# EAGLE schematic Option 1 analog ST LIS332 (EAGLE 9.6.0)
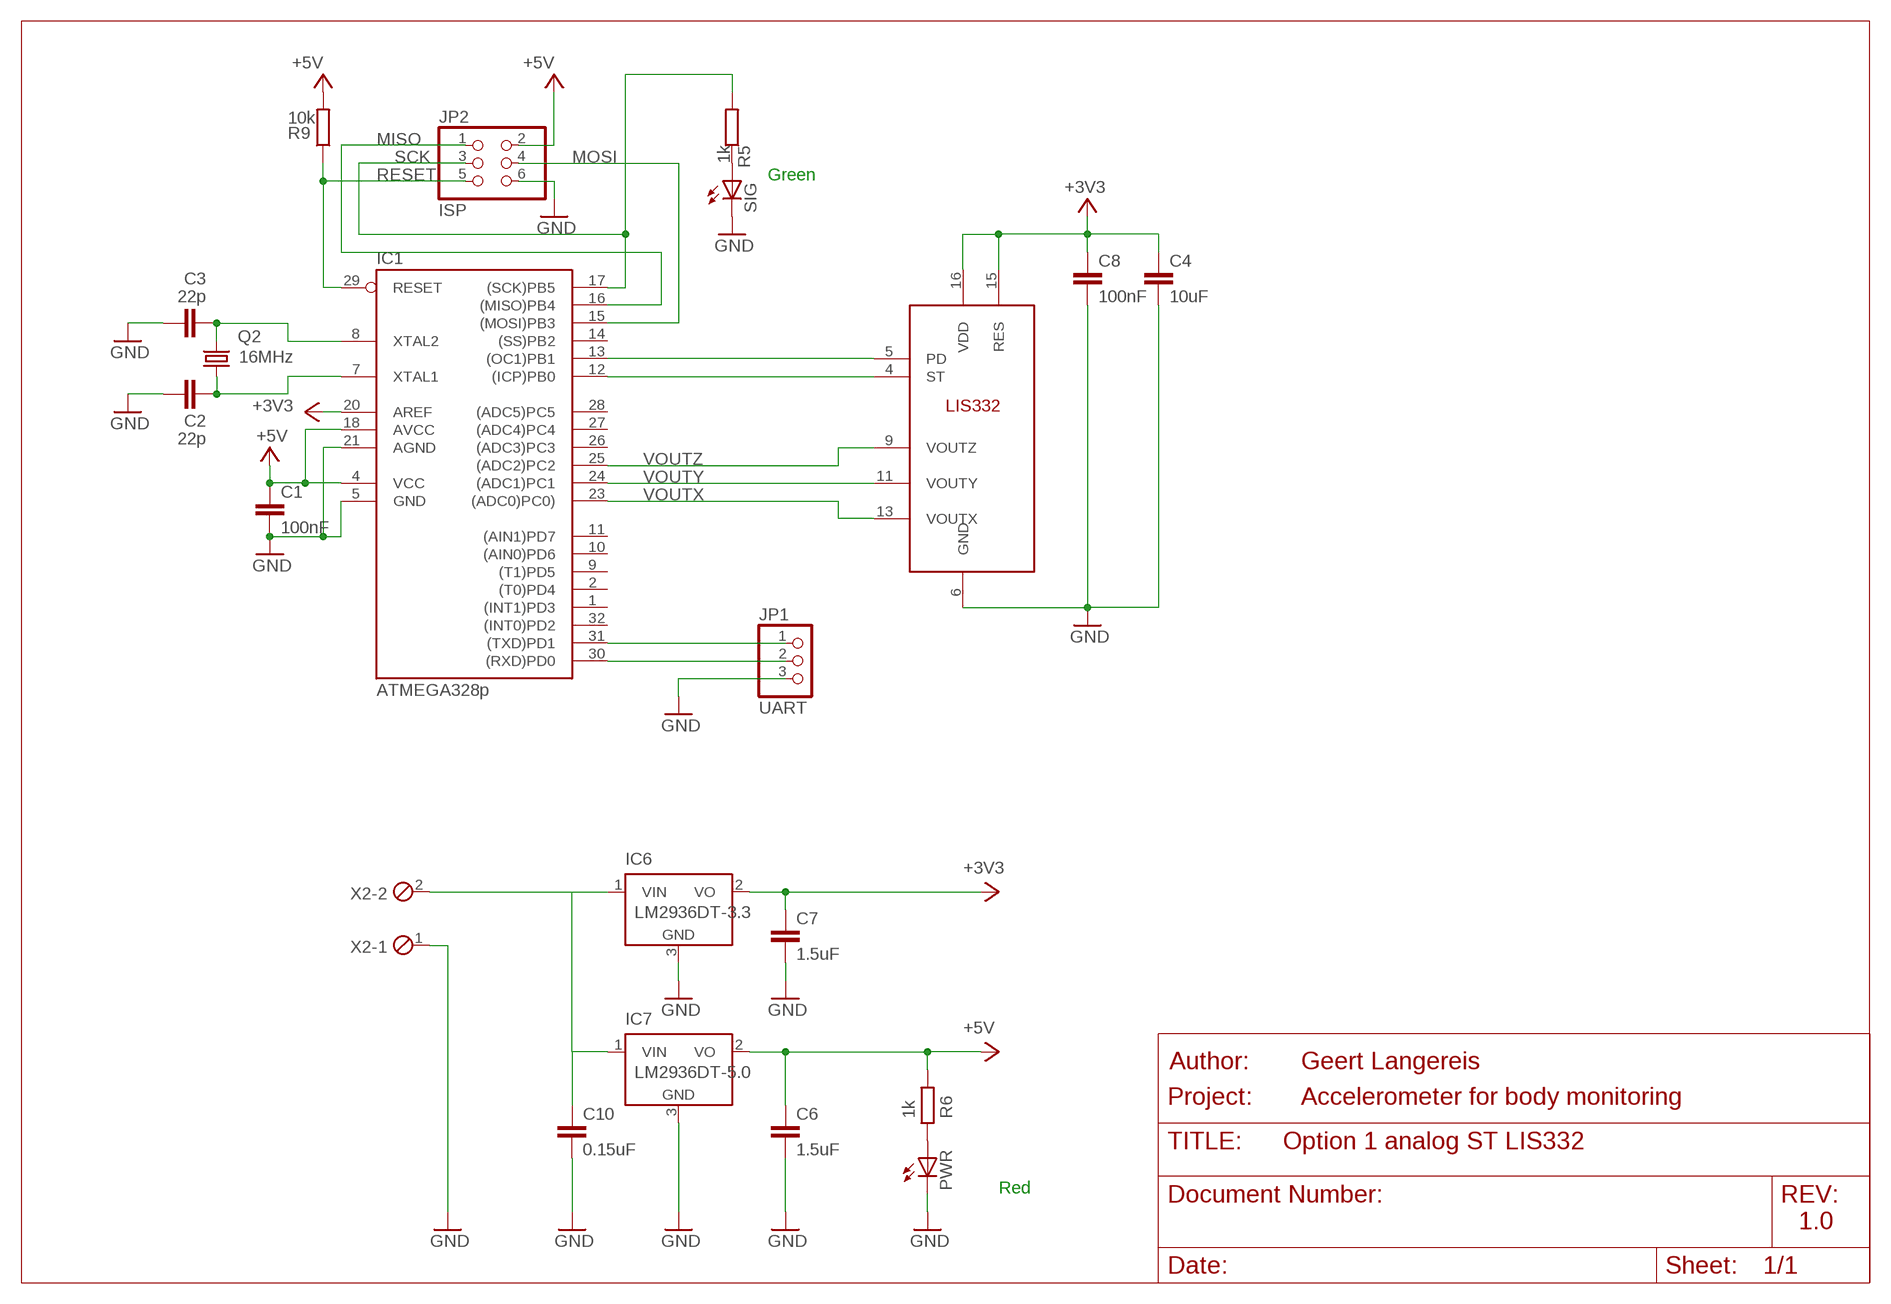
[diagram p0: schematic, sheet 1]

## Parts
C1  100nF  C5/3.5  [C5B3.5]
C2  22p  C2.5/2  [C2.5-2]
C3  22p  C2.5/2  [C2.5-2]
C4  10uF  C-EU050-030X075  [C050-030X075]
C6  1.5uF  C5/3.5  [C5B3.5]
C7  1.5uF  C5/3.5  [C5B3.5]
C8  100nF  C-EU050-030X075  [C050-030X075]
C10  0.15uF  C5/3.5  [C5B3.5]
IC1  ATMEGA328p  AT90S4433A  [TQFP32-08]
IC3  LIS332AR  [QFN-16]
IC6  LM2936DT-3.3  [TO252]
IC7  LM2936DT-5.0  [TO252]
JP1  UART  PINHD-1X3  [1X03]
JP2  ISP  PINHD-2X3  [2X03]
PWR  LED3MM  [LED3MM]
Q2  16MHz  CRYTALHC49S  [HC49/S]
R5  1k  R-EU_0204/7  [0204/7]
R6  1k  R-EU_0204/7  [0204/7]
R9  10k  R-EU_0204/7  [0204/7]
SIG  LED3MM  [LED3MM]
X2  MPT2  [2POL254]

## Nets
+3V3 [usbvcc]: C4.1 C7.1 C8.1 IC1.20(AREF) IC3.15(RES) IC3.16(VDD) IC6.2(VO)
+5V: JP2.2 R9.2
+9V [usbvcc]: C10.1 IC6.1(VIN) IC7.1(VIN) X2.2
GND [gnd]: C1.2 C2.1 C3.1 C4.2 C6.2 C7.2 C8.2 C10.2 IC1.5(GND) IC1.21(AGND) IC3.6(GND) IC6.3(GND) IC7.3(GND) JP1.3 JP2.6 PWR.K(C) SIG.K(C) X2.1
MISO: IC1.16((MISO)PB4) JP2.1
MOSI: IC1.15((MOSI)PB3) JP2.4
N$1: IC1.31((TXD)PD1) JP1.1
N$2: IC1.30((RXD)PD0) JP1.2
N$3: PWR.A R6.2
N$4: R5.1 SIG.A
N$6: C2.2 IC1.7(XTAL1) Q2.1
N$7: C3.2 IC1.8(XTAL2) Q2.2
N$8: IC1.13((OC1)PB1) IC3.5(PD)
N$9: IC1.12((ICP)PB0) IC3.4(ST)
RESET [usbvcc]: IC1.29(RESET) JP2.5 R9.1
SCK: IC1.17((SCK)PB5) JP2.3 R5.2
VCC: C1.1 C6.1 IC1.4(VCC) IC1.18(AVCC) IC7.2(VO) R6.1 ; supply symbol labelled +5V
VOUTX: IC1.23((ADC0)PC0)) IC3.13(VOUTX)
VOUTY: IC1.24((ADC1)PC1) IC3.11(VOUTY)
VOUTZ: IC1.25((ADC2)PC2) IC3.9(VOUTZ)
Unconnected: IC1.1((INT1)PD3) IC1.2((T0)PD4) IC1.9((T1)PD5) IC1.10((AIN0)PD6) IC1.11((AIN1)PD7) IC1.14((SS)PB2) IC1.26((ADC3)PC3) IC1.27((ADC4)PC4) IC1.28((ADC5)PC5) IC1.32((INT0)PD2)

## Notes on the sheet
- Green
- Geert Langereis
- Accelerometer for body monitoring
- Red
- 1.0

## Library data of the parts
C1-C3 C6 C7 C10 = capacitor-wima:C: CAPACITOR
C4 C8 = resistor:C-EU: CAPACITOR, European symbol
IC1 = atmel:AT90S4433: MICROCONTROLLER 4 Kbytes FLASH 128 bytes SRAM 256 bytes EEPROM UART 6-channel 10 bit ADC; OC_FARNELL: unknown; OC_NEWARK: unknown
IC3 = Geert-library:LIS332AR: 3-Axis, Analog Accelerometer (ST)
IC6 = national-semiconductor:LM2936?*: Ultra-Low Quiescent Current LDO Voltage Regulator Source: Data sheet; MPN: LM2936DT-3.3.; OC_FARNELL: 1286863; OC_NEWARK: 26M0361
IC7 = national-semiconductor:LM2936?*: Ultra-Low Quiescent Current LDO Voltage Regulator Source: Data sheet; MF: NATIONAL SEMICONDUCTOR; MPN: LM2936DT-5.0/NOPB; OC_FARNELL: 1286864; OC_NEWARK: 41K4501
JP1 = pinhead:PINHD-1X3: PIN HEADER
JP2 = pinhead:PINHD-2X3: PIN HEADER
PWR SIG = led:LED: LED
Q2 = crystal:CRYTAL: CRYSTAL
R5 R6 R9 = resistor:R-EU_: RESISTOR, European symbol
X2 = con-phoenix-254:MPT2: PHOENIX CONNECTOR; OC_FARNELL: unknown; OC_NEWARK: unknown

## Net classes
0 default: width 0.254 mm, drill 0.305 mm, clearance 0.152 mm
1 power: width 0.61 mm, drill 0.508 mm, clearance 0.152 mm
2 gnd: width 0.305 mm, drill 0.508 mm, clearance 0.152 mm
3 usbvcc: width 0.508 mm, drill 0.508 mm, clearance 0.152 mm
4 aref: width 0.406 mm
